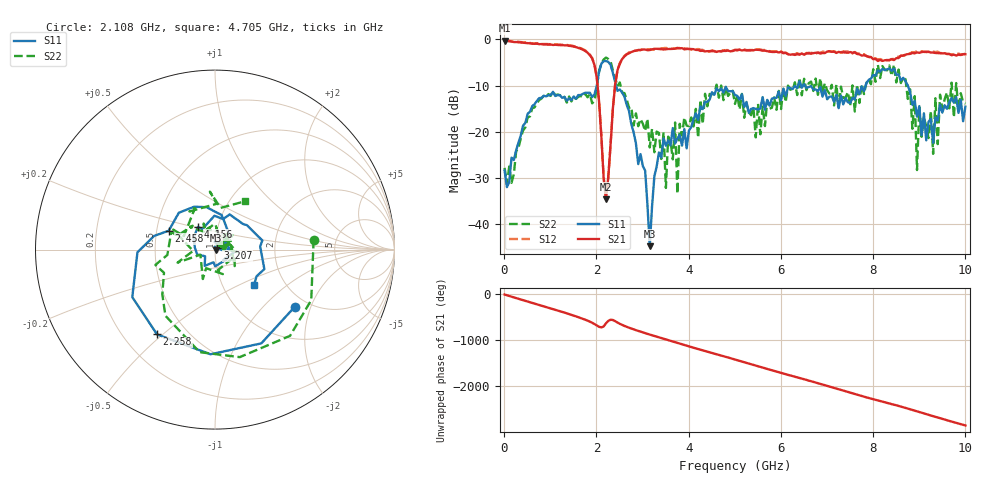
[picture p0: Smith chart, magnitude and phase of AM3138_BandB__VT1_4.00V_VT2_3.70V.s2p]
! Date/Time: Tue, Nov 13, 2018 4:40 PM
! Network Analyzer: Agilent Technologies E8364B Rev: A.07.50.67
! Sweep from 0.010 to 10.000 GHz, 201 Points, Sweep Type: LIN
! Power Supply: 4.001 V, 0.000 A
# Hz S DB R 50
!freq MagS11 AngS11 MagS21 AngS21 MagS12 AngS12 MagS22 AngS22
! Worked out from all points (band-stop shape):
!   201 points, 10 MHz to 10 GHz, reference 50 ohm
!   highest |S21| = -0.27 dB at 10 MHz (marker M1); lowest = -34.6 dB at 2.208 GHz (marker M2)
!   |S21| within 3 dB of the highest: start of sweep to 1.847 GHz; 2.653 GHz to 6.19 GHz (3.537 GHz wide, 80 % of centre)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
!   lowest |S11| = -44.7 dB at 3.157 GHz (marker M3), VSWR 1.01, Z = 50.4 - j0.447 ohm
!   |S11| at or under -10 dB: start of sweep to 2.009 GHz; 2.429 GHz to 6.371 GHz (3.943 GHz wide, 89.6 % of centre); 6.524 GHz to 7.837 GHz (1.313 GHz wide, 18.3 % of centre)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
!   |S22| runs from -33.4 to -3.9 dB; largest |S21 - S12| = 0.031
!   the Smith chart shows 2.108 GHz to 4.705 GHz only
!   S11 on the Smith chart (normalised r, x): 2.108 GHz: 1.71, -1.55; 2.258 GHz: 0.34, -0.48; 2.458 GHz: 0.58, +0.13; 3.207 GHz: 1.03, +0.02; 4.156 GHz: 0.80, +0.21; 4.705 GHz: 1.40, -0.61
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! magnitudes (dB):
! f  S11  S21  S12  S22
! 10 MHz  -28.4  -0.3  -0.2  -27.8
! 1.708 GHz  -11.8  -2.2  -2.1  -12.5
! 2.108 GHz  -5.2  -21.0  -20.9  -5.2
! 2.208 GHz  -4.7  -34.6  -34.2  -3.9
! 2.258 GHz  -4.8  -29.8  -29.7  -4.2
! 2.458 GHz  -11.1  -6.6  -6.6  -10.1
! 3.157 GHz  -44.7  -2.3  -2.1  -23.4
! 3.207 GHz  -36.1  -2.2  -2.2  -19.3
! 3.357 GHz  -24.4  -2.1  -2.0  -20.2
! 3.507 GHz  -23.0  -2.1  -1.8  -32.1
! 3.706 GHz  -22.5  -2.0  -2.0  -18.0
! 3.756 GHz  -21.5  -1.8  -1.9  -33.4
! 3.806 GHz  -20.6  -1.9  -1.8  -18.2
! 4.156 GHz  -16.0  -2.3  -2.1  -15.0
! 4.705 GHz  -10.6  -2.6  -2.5  -10.0
! 5.005 GHz  -12.0  -2.3  -2.2  -14.0
! 6.703 GHz  -10.8  -3.0  -2.9  -11.1
! 8.352 GHz  -6.3  -4.5  -4.5  -5.6
! 8.901 GHz  -13.3  -3.0  -2.8  -12.3
! 8.951 GHz  -16.7  -2.8  -2.6  -28.3
! 9.001 GHz  -14.4  -2.9  -2.6  -14.7
! 10 GHz  -14.5  -3.2  -3.1  -13.9
